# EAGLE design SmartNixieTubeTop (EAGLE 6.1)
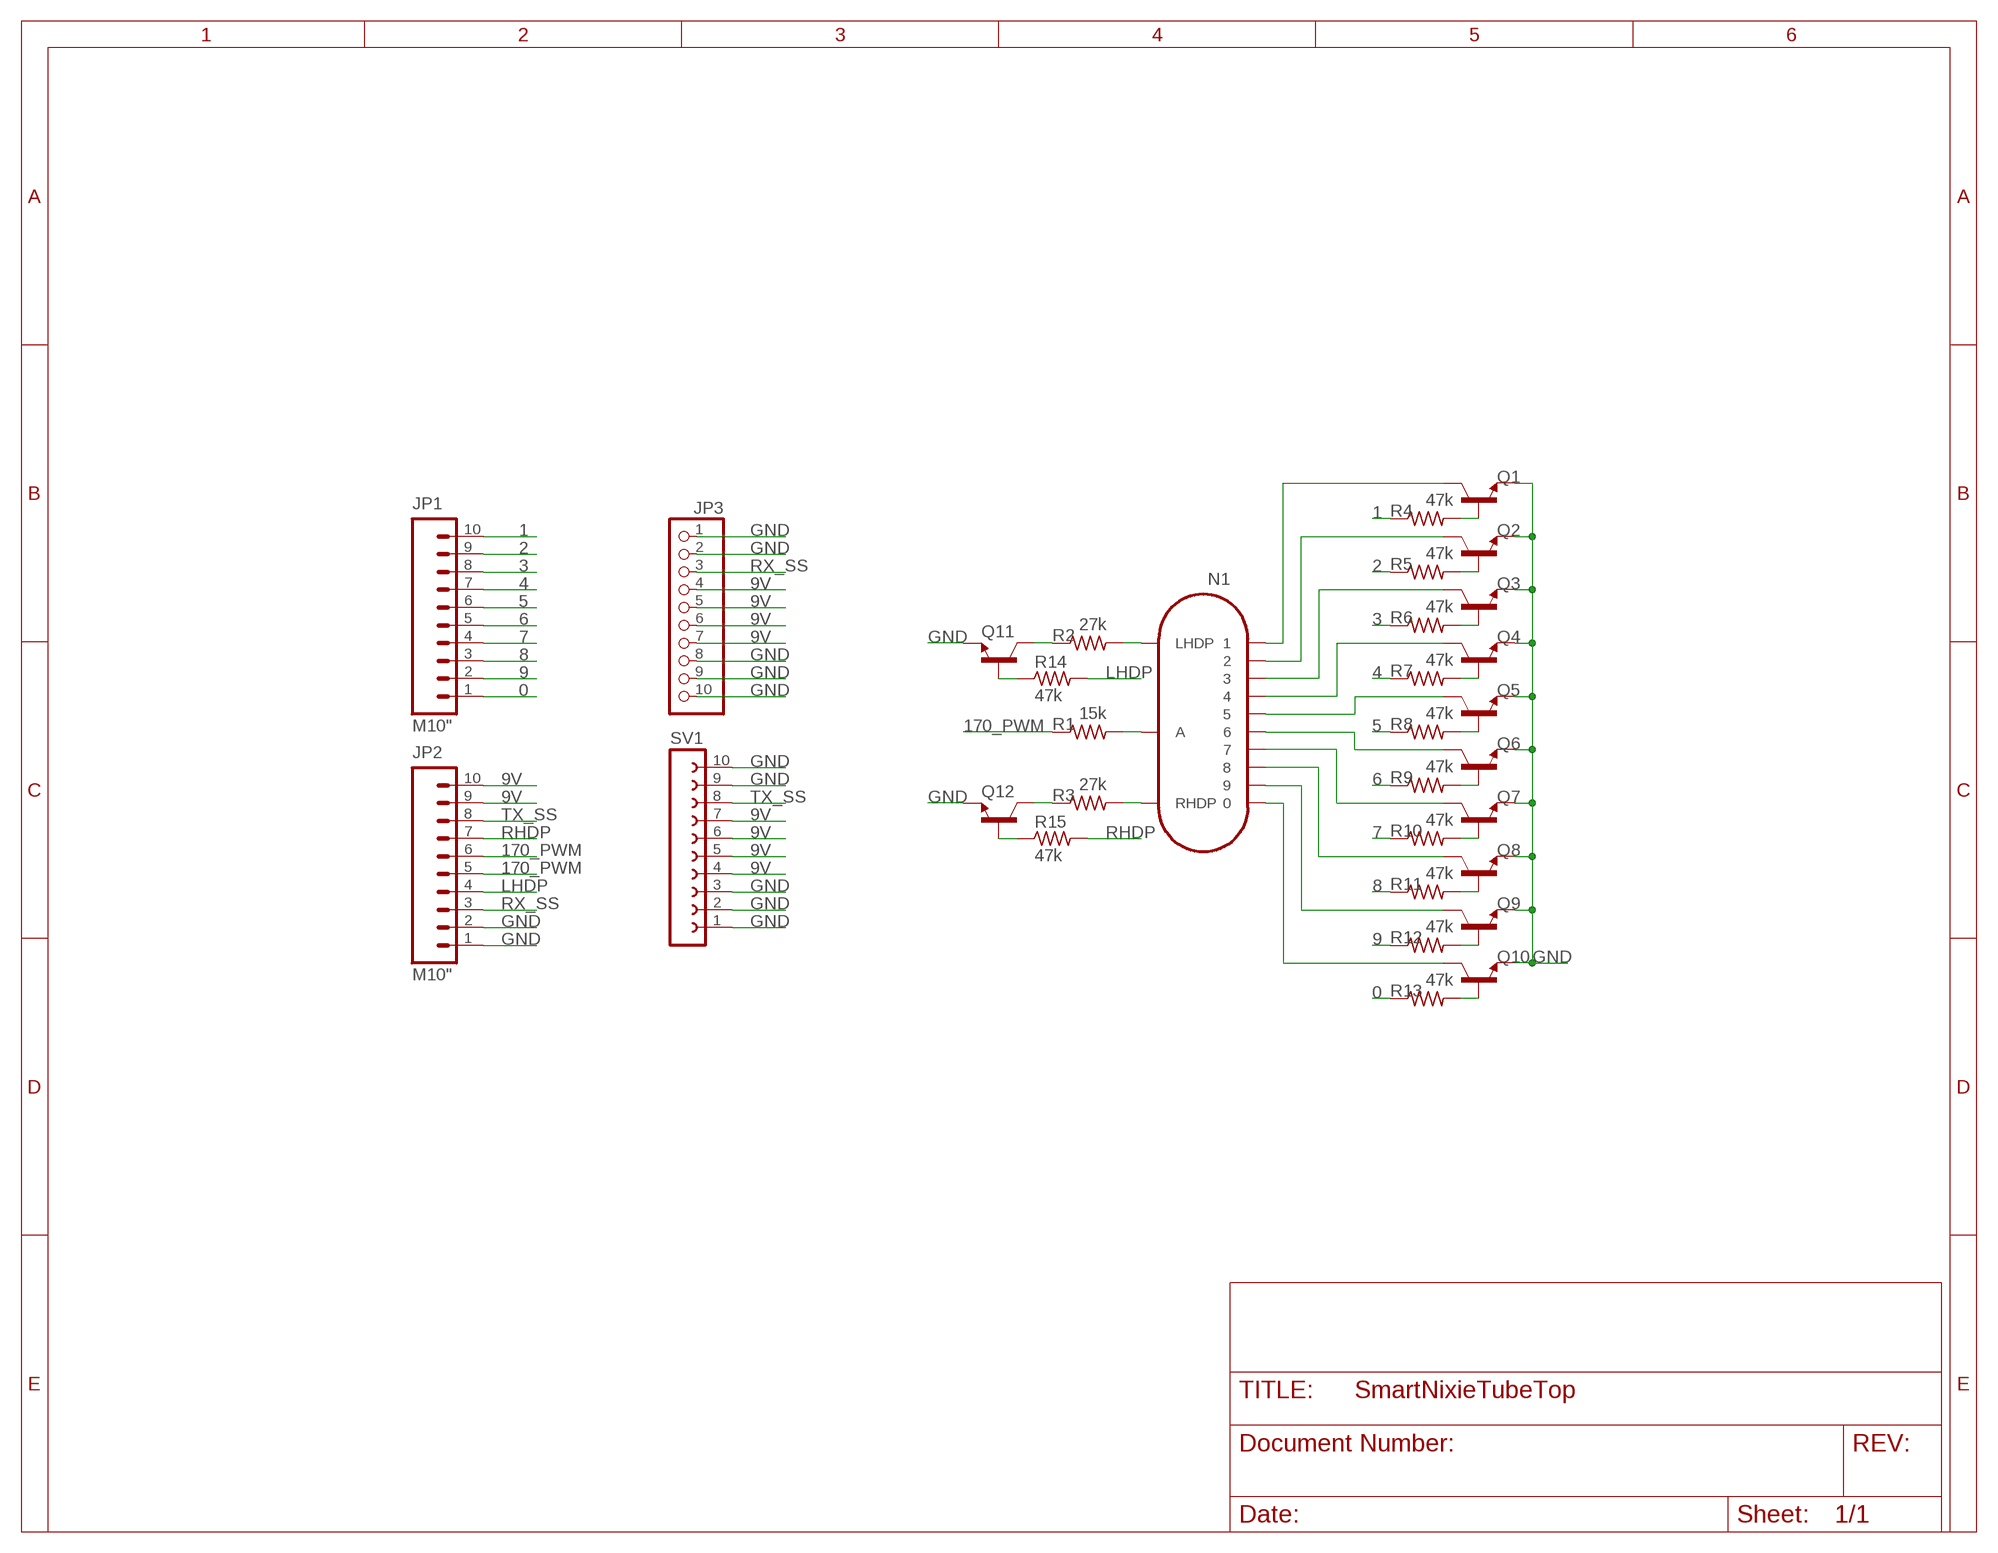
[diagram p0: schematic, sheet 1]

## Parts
JP1  M10"  [1X10]
JP2  M10"  [1X10]
JP3  PINHD-1X10/90  [1X10/90]
N1  IN-14  [IN-14]
Q1  TRANSISTOR_NPNTO-92-AMMO  [TO-92-AMMO]
Q2  TRANSISTOR_NPNTO-92-AMMO  [TO-92-AMMO]
Q3  TRANSISTOR_NPNTO-92-AMMO  [TO-92-AMMO]
Q4  TRANSISTOR_NPNTO-92-AMMO  [TO-92-AMMO]
Q5  TRANSISTOR_NPNTO-92-AMMO  [TO-92-AMMO]
Q6  TRANSISTOR_NPNTO-92-AMMO  [TO-92-AMMO]
Q7  TRANSISTOR_NPNTO-92-AMMO  [TO-92-AMMO]
Q8  TRANSISTOR_NPNTO-92-AMMO  [TO-92-AMMO]
Q9  TRANSISTOR_NPNTO-92-AMMO  [TO-92-AMMO]
Q10  TRANSISTOR_NPNTO-92-AMMO  [TO-92-AMMO]
Q11  TRANSISTOR_NPNTO-92-AMMO  [TO-92-AMMO]
Q12  TRANSISTOR_NPNTO-92-AMMO  [TO-92-AMMO]
R1  15k  R-US_0204/5  [0204/5]
R2  27k  R-US_0204/5  [0204/5]
R3  27k  R-US_0204/5  [0204/5]
R4  47k  R-US_0204/5  [0204/5]
R5  47k  R-US_0204/5  [0204/5]
R6  47k  R-US_0204/5  [0204/5]
R7  47k  R-US_0204/5  [0204/5]
R8  47k  R-US_0204/5  [0204/5]
R9  47k  R-US_0204/5  [0204/5]
R10  47k  R-US_0204/5  [0204/5]
R11  47k  R-US_0204/5  [0204/5]
R12  47k  R-US_0204/5  [0204/5]
R13  47k  R-US_0204/5  [0204/5]
R14  47k  R-US_0204/5  [0204/5]
R15  47k  R-US_0204/5  [0204/5]
SV1  FE10W  [FE10W]

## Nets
0: JP1.1 R13.1
1: JP1.10 R4.1
2: JP1.9 R5.1
3: JP1.8 R6.1
4: JP1.7 R7.1
5: JP1.6 R8.1
6: JP1.5 R9.1
7: JP1.4 R10.1
8: JP1.3 R11.1
9: JP1.2 R12.1
9V: JP2.9 JP2.10 JP3.4 JP3.5 JP3.6 JP3.7 SV1.4 SV1.5 SV1.6 SV1.7
170_PWM: JP2.5 JP2.6 R1.1
GND: JP2.1 JP2.2 JP3.1 JP3.2 JP3.8 JP3.9 JP3.10 Q1.1(E) Q2.1(E) Q3.1(E) Q4.1(E) Q5.1(E) Q6.1(E) Q7.1(E) Q8.1(E) Q9.1(E) Q10.1(E) Q11.1(E) Q12.1(E) SV1.1 SV1.2 SV1.3 SV1.9 SV1.10
LHDP: JP2.4 R14.2
N$1: N1.5 Q5.3(C)
N$2: N1.6 Q6.3(C)
N$3: N1.1 Q1.3(C)
N$4: N1.2 Q2.3(C)
N$5: N1.3 Q3.3(C)
N$6: N1.4 Q4.3(C)
N$7: N1.A R1.2
N$8: Q11.2(B) R14.1
N$9: N1.0 Q10.3(C)
N$10: N1.9 Q9.3(C)
N$11: N1.8 Q8.3(C)
N$12: N1.7 Q7.3(C)
N$13: Q12.2(B) R15.1
N$14: Q1.2(B) R4.2
N$15: Q2.2(B) R5.2
N$16: Q3.2(B) R6.2
N$17: Q4.2(B) R7.2
N$18: Q5.2(B) R8.2
N$19: Q6.2(B) R9.2
N$20: Q7.2(B) R10.2
N$21: N1.LHDP R2.2
N$22: Q11.3(C) R2.1
N$23: N1.RHDP R3.2
N$24: Q12.3(C) R3.1
N$25: Q8.2(B) R11.2
N$26: Q9.2(B) R12.2
N$27: Q10.2(B) R13.2
RHDP: JP2.7 R15.2
RX_SS: JP2.3 JP3.3
TX_SS: JP2.8 SV1.8

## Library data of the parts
JP1 JP2 = SparkFun-Connectors_tyler:M10: Header 10 Standard 10-pin 0.1" header. Use with straight break away headers (SKU : PRT-00116), right angle break away headers (PRT-00553), swiss pins (PRT-00743), machine pins (PRT-00117), and female headers (PRT-00115).
JP3 = pinhead:PINHD-1X10: PIN HEADER
N1 = russian-nixies:IN-14: IN-14: medium numeric frontview nixie tube
Q1-Q12 = SparkFun-DiscreteSemi:TRANSISTOR_NPN: Generic NPN BJT. MMBT2222 is the common NPN we use. Double check against datasheet- not all devices are the same!
R1-R15 = resistor:R-US_: RESISTOR, American symbol
SV1 = con-lsta_tyler:FE10W: FEMALE HEADER; OC_FARNELL: unknown; OC_NEWARK: unknown

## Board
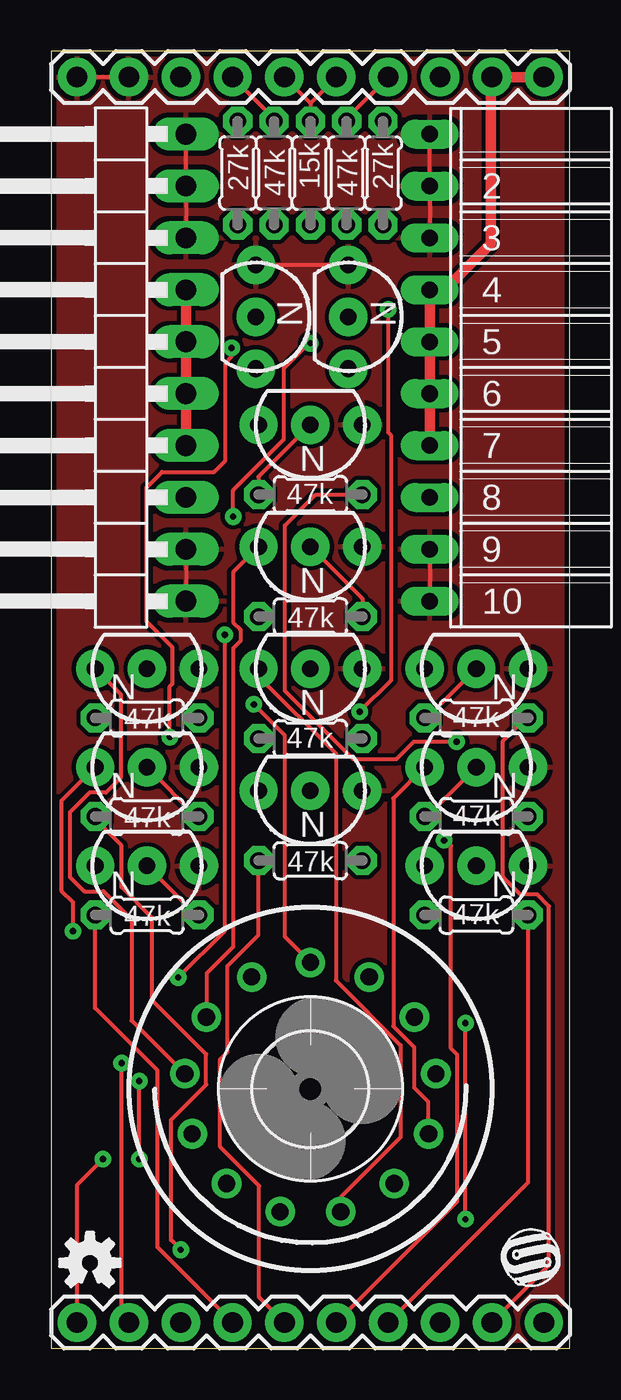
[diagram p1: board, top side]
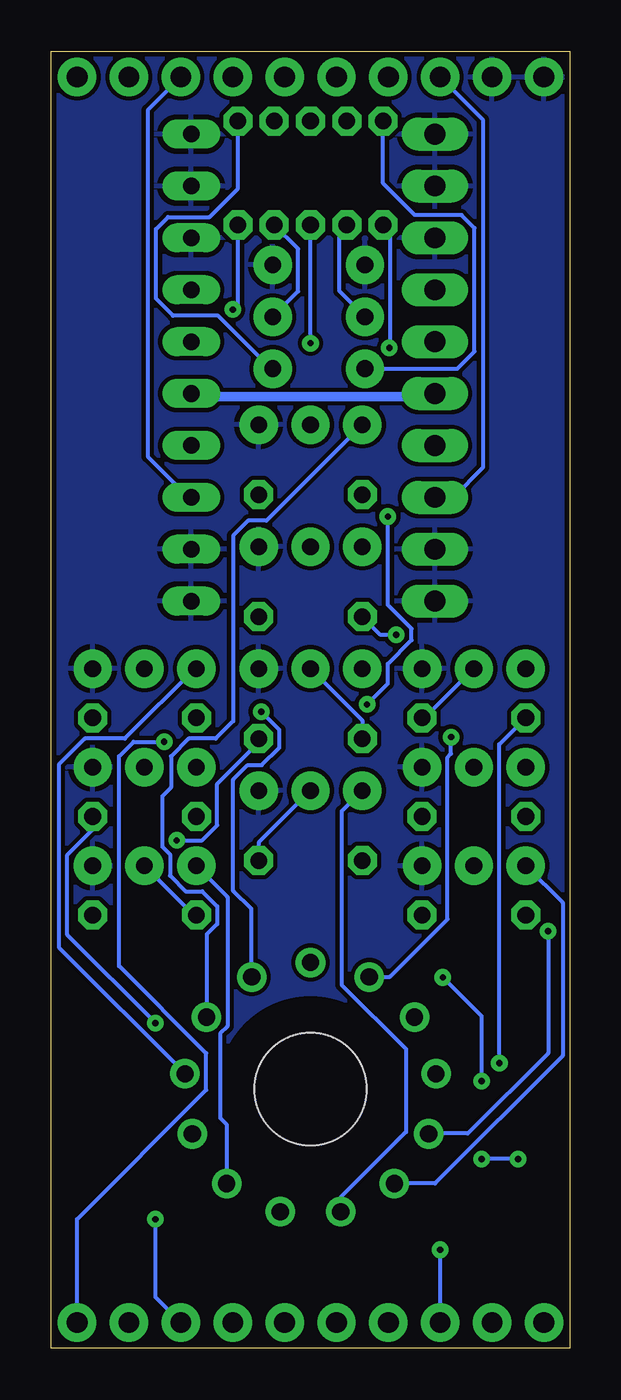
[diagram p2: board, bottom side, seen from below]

Size 25.41 x 63.5 mm. Coordinates in mm from the lower left corner, seen from the top.
Outline: 0,0 25.41,0 25.41,63.5 0,63.5 0,0
Copper layers (1*16): Top 0.035mm / dielectric 1.5mm / Bottom 0.035mm
Design rules: minimum track width 8mil, minimum drill 12mil, track to track 8mil, track to pad 8mil, pad to pad 8mil, via to via 8mil, smd to smd 8mil, copper to edge 10mil, drill to drill 6mil, minimum pad ring 12mil, minimum via ring 10mil, stop-mask expansion 4mil, vias tented up to drill 25mil, thermal gap 10mil

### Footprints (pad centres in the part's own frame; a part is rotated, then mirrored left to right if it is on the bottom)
1X10 = drill 1.016 pad 1.88: 1 0,0; 2 2.54,0; 3 5.08,0; 4 7.62,0; 5 10.16,0; 6 12.7,0; 7 15.24,0; 8 17.78,0; 9 20.32,0; 10 22.86,0
1X10/90 = drill 1.016 long: 1 -11.43,-3.81; 2 -8.89,-3.81; 3 -6.35,-3.81; 4 -3.81,-3.81; 5 -1.27,-3.81; 6 1.27,-3.81; 7 3.81,-3.81; 8 6.35,-3.81; 9 8.89,-3.81; 10 11.43,-3.81
IN-14 = drill 0.84: 0 5.094,-3.516; 1 -5.094,-3.516; 2 -6.145,-0.746; 3 -5.788,2.195; 4 -4.105,4.633; 5 -1.481,6.01; 6 1.481,6.01; 7 4.105,4.633; 8 5.788,2.195; 9 6.145,-0.746; A 0,-6.19; LHDP 2.877,-5.481; RHDP -2.877,-5.481
TO-92-AMMO = drill 0.813 pad 1.88: 1 -2.54,0; 2 0,0; 3 2.54,0
0204/5 = drill 0.813 octagon: 1 -2.54,0; 2 2.54,0
FE10W = drill 0.813 long: 1 -11.43,0; 2 -8.89,0; 3 -6.35,0; 4 -3.81,0; 5 -1.27,0; 6 1.27,0; 7 3.81,0; 8 6.35,0; 9 8.89,0; 10 11.43,0
5,5 = hole 5.5: 0,0

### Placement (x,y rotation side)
JP1  1.27,1.27 0 top
JP2  1.27,62.23 0 top
JP3  2.79,48.01 90 top
N1  12.7,12.7 180 top
Q1  12.7,45.21 180 top
Q2  20.83,33.27 180 top
Q3  20.83,28.45 180 top
Q4  20.83,23.62 180 top
Q5  12.7,33.27 180 top
Q6  12.7,27.3 180 top
Q7  4.7,23.62 180 top
Q8  4.7,28.45 180 top
Q9  4.7,33.27 180 top
Q10  12.7,39.24 180 top
Q11  10.03,50.5 270 top
Q12  14.55,50.5 270 top
R1  12.7,57.53 270 top
R2  9.14,57.53 270 top
R3  16.26,57.53 270 top
R4  12.7,41.78 180 top
R5  20.83,30.86 180 top
R6  20.83,26.04 180 top
R7  20.83,21.21 180 top
R8  12.7,29.84 180 top
R9  12.7,23.88 0 top
R10  4.7,21.21 0 top
R11  4.7,26.04 0 top
R12  4.7,30.86 0 top
R13  12.7,35.81 0 top
R14  10.92,57.53 90 top
R15  14.48,57.53 90 top
SV1  18.54,48.01 270 top
U$1  [5,5]  12.7,12.7 0 top
U$2  [OSHW-LOGO-S]  1.91,4.19 0 top
U$3  [SWITCHMODE_LOGO_S]  21.89,2.82 0 top

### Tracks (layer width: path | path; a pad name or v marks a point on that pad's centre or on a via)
0  (via drill 0.3)
  Top 0.203: JP1.1 1.27,8 v2.54,9.27 | v4.32,9.27 v4.32,13.08 | v6.22,18.16 8.51,20.45 v8.51,34.92
  Bottom 0.203: v2.54,9.27 v4.32,9.27 | v4.32,13.08 4.32,16.26 v6.22,18.16 | v8.51,34.92 9.27,34.92 R13.1
1  (via drill 0.3)
  Top 0.203: R4.1 12.95,41.78 11.46,40.28 11.46,32.18 14.81,28.83 16.89,28.83 17.75,29.69 v19.86,29.69
  Bottom 0.203: v19.86,29.69 21.36,29.69 22.07,28.98 22.07,18.72 17.8,14.45 17.8,12.65 24.13,6.33 JP1.10
2
  Top 0.203: R5.1 23.37,30.99 22.12,29.74 22.12,23.09 22.99,22.23 23.8,22.23 24.38,21.64 24.38,4.06 JP1.9
3  (via drill 0.3)
  Top 0.203: v20.3,6.33 v20.3,15.93
  Bottom 0.203: R6.1 23.37,25.4 24.61,24.16 24.61,20.24 v20.3,15.93 | v20.3,6.33 20.3,2.52 JP1.8
4
  Top 0.203: R7.1 23.37,8.13 JP1.7
5  (via drill 0.3)
  Top 0.203: v19.25,24.87 19.25,24.94 19.58,24.61 19.58,14.68 19.89,14.38 19.89,7.19 JP1.6
  Bottom 0.203: R8.1 15.24,29.67 17.27,27.64 17.27,25.6 18.01,24.87 v19.25,24.87
6
  Top 0.203: R9.1 10.16,20.24 8.64,18.72 8.64,14.5 8.28,14.15 8.28,9.86 10.19,7.95 10.19,2.52 JP1.5
7
  Top 0.203: R10.1 2.16,16.66 5.21,13.61 5.21,4.95 JP1.4
8  (via drill 0.3)
  Top 0.203: R11.1 2.16,25.91 3.45,24.61 3.45,22.58 4.95,21.08 4.95,17.04 7.59,14.4 7.59,12.9 5.87,11.18 5.87,5.31 v6.35,4.83
  Bottom 0.203: JP1.3 v6.35,4.83
9  (via drill 0.3)
  Top 0.203: v3.45,13.97 3.45,1.63 JP1.2
  Bottom 0.203: R12.1 3.45,29.57 v3.45,13.97
9V
  Top 0.203: 21.54,62.15 JP2.9
  Top 0.508: JP3.4 JP3.5 JP3.6 JP3.7 | JP2.10 JP2.9 | SV1.7 SV1.6 SV1.5 SV1.4 19.28,51.82 21.54,54.08 21.54,62.15
  Bottom 0.203: JP3.5 6.68,46.74 6.71,46.71 6.6,46.71 6.71,46.58 | 18.39,46.58 18.49,46.71 18.52,46.71 SV1.6
  Bottom 0.457: 18.39,46.58 6.71,46.58
170_PWM
  Top 0.203: 12.7,60.96 R1.1 | JP2.5 12.7,60.96 | 12.7,60.96 JP2.6
GND
  Top 0.203: JP2.1 JP2.2 3.89,62.18 | SV1.3 SV1.2 SV1.1 | JP3.8 JP3.9 JP3.10 6.55,59.51 | Q11.1 Q12.1 | SV1.9 SV1.10 | JP3.2 JP3.1
  pour Bottom (isolate 0.203): 0,0 25.4,0 25.4,63.5 0,63.5
  pour Top (isolate 0.203): 0,0 25.4,0 25.4,63.5 0,63.5
LHDP
  Top 0.203: R14.2 10.92,60.2 JP2.4
N$1
  Top 0.203: Q5.3 10.16,32.89 13.95,29.11 13.95,18.01 17.12,14.83 17.12,10.34 14.2,7.42 14.2,6.71 N1.5
N$2
  Bottom 0.203: Q6.3 11.18,26.29 11.18,17.8 8.03,14.66 8.03,10.59 11.2,7.42 11.2,6.71 N1.6
N$3
  Bottom 0.203: Q1.3 14.86,40.51 15.75,40.51 16.48,39.78 16.48,30.71 17.35,29.84 18.67,29.84 19.53,28.98 19.53,27.46 19.96,27.03 19.96,24.56 19.58,24.18 19.58,23.14 18.82,22.38 18.01,22.38 17.27,21.64 17.27,20.78 17.78,20.27 17.78,16.23 N1.1
N$4
  Bottom 0.203: Q2.3 18.36,33.27 21.79,29.84 23.75,29.84 25.02,28.57 25.02,19.63 18.85,13.46 N1.2
N$5
  Top 0.203: Q3.3 16.76,26.92 16.76,15.77 17.78,14.76 17.78,12.78 18.47,12.09 18.47,10.52 N1.3
N$6
  Bottom 0.203: Q4.3 16.76,22.1 16.76,15.77 17.12,15.42 17.12,11.28 16.82,10.97 16.82,8.08 N1.4
N$7  (via drill 0.3)
  Top 0.203: v12.7,49.2 12.7,49.28 11.4,47.98 11.4,44.5 8.91,42.01 v8.91,40.72 | v9.93,31.52 11.46,30 11.46,20.14 N1.A
  Bottom 0.203: v12.7,49.2 R1.2 | v8.91,40.72 8.91,36.4 7.75,35.23 7.75,34.67 8.91,33.5 8.91,32.54 v9.93,31.52
N$8
  Bottom 0.203: R14.1 10.92,54.94 11.28,54.59 11.28,51.74 Q11.2
N$9
  Top 0.203: Q10.3 8.91,38 8.91,35.53 9.27,35.18 9.27,34.62 8.91,34.27 8.91,19.66 7.62,18.36 7.62,16.23 N1.0
N$10
  Top 0.203: Q9.3 3.4,32.03 3.4,27.91 2.69,27.2 1.88,27.2 0.91,26.24 0.91,23.09 1.63,22.38 2.56,22.38 3.94,21.01 3.94,16.05 6.55,13.44 6.55,13.46 N1.9
N$11  (via drill 0.3)
  Top 0.203: v1.07,20.42 1.07,21.84 0.51,22.4 0.51,26.8 Q8.3
  Bottom 0.203: v1.07,20.42 1.07,14.45 5,10.52 6.91,10.52 N1.8
N$12
  Bottom 0.203: Q7.3 0.36,21.82 0.36,14.33 6.6,8.08 8.59,8.08 N1.7
N$13
  Bottom 0.203: R15.1 13.31,53.82 13.31,51.74 Q12.2
N$14
  Top 0.203: R4.2 10.16,42.67 Q1.2
N$15
  Top 0.203: R5.2 18.41,30.86 Q2.2
N$16
  Top 0.203: R6.2 18.41,26.04 Q3.2
N$17
  Bottom 0.203: R7.2 18.41,21.21 Q4.2
N$18
  Bottom 0.203: R8.2 10.16,30.73 Q5.2
N$19
  Bottom 0.203: R9.2 15.24,24.77 Q6.2
N$20
  Top 0.203: R10.2 7.11,21.21 Q7.2
N$21  (via drill 0.3)
  Top 0.203: v8.84,48.97 8.84,48.54 8.53,48.23 8.53,43.46 7.98,42.9 5.44,42.9 4.67,42.14 4.67,35.59 5.94,34.31 5.94,32.54 5.82,32.41 v5.82,29.92
  Bottom 0.203: R2.2 9.14,54.94 8.79,54.59 8.79,49.02 v8.84,48.97 | v5.82,29.92 5.82,29.11 5.99,28.93 5.99,21.01 8.81,18.19 9.8,18.19 N1.LHDP
N$22
  Bottom 0.203: R2.1 9.14,57.02 7.59,55.47 5.31,55.47 4.67,54.84 4.67,48.79 5.51,47.95 Q11.3
N$23  (via drill 0.3)
  Top 0.203: v16.51,50.85 16.51,44.83 16.66,44.68 16.66,32.72 v15.11,31.17
  Bottom 0.203: R3.2 16.26,51.1 v16.51,50.85 | v15.11,31.17 14.22,30.28 14.22,29.41 15.09,28.55 15.77,28.55 16.48,27.84 16.48,22.4 15.6,21.51 15.6,18.19 N1.RHDP
N$24
  Bottom 0.203: R3.1 16.26,56.77 17.65,55.37 19.68,55.37 20.27,54.79 20.27,51.38 19.43,50.55 17.22,50.55 14.63,47.95 Q12.3
N$25
  Top 0.203: R11.2 7.11,26.04 Q8.2
N$26
  Bottom 0.203: R12.2 7.11,30.86 Q9.2
N$27
  Top 0.203: R13.2 15.24,36.7 Q10.2
RHDP
  Top 0.203: R15.2 14.48,60.2 JP2.7
RX_SS
  Bottom 0.203: JP3.3 5.71,41.66 4.27,43.1 4.27,60.15 JP2.3
TX_SS
  Bottom 0.203: SV1.8 18.54,41.53 20.68,43.66 20.68,60.6 JP2.8

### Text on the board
tPlace: N | N | N | N | N | N | N | N | N | N | N | N
tValues: 3

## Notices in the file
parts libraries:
SparkFun-DiscreteSemi: Licensing: CC v3.0 Share-Alike You are welcome to use this library for commercial purposes.
